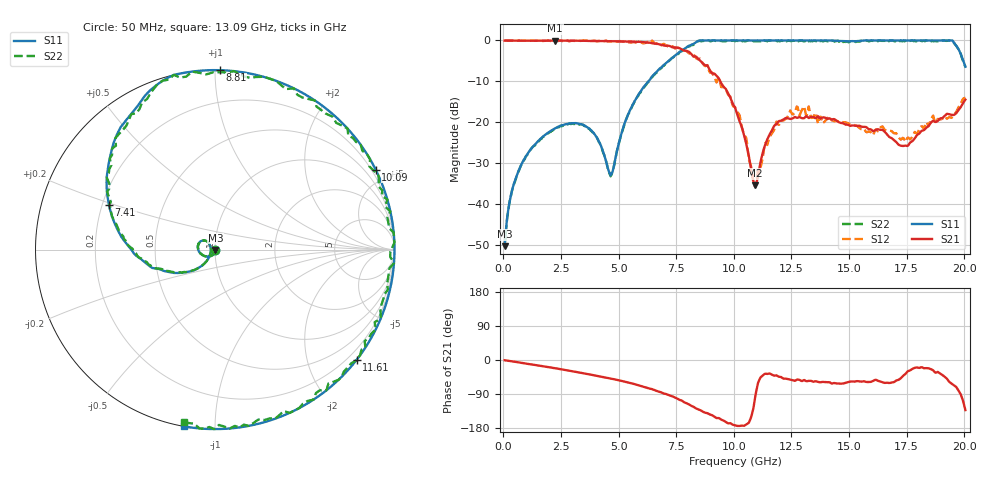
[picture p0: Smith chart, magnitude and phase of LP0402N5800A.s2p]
!	AVX	THIN	FILM	OPERATION
!	0402	SIZE	LOW	PASS	FILTER	P/N	LP0402N5800ANTR
!	Created	December	2017
!	Network	Analyzer	HP8720E	S.07.64:	"Feb23,"	2000	Serial	No.US39172382
#	MHz	S	dB	R	50
!	Frq	S11(dB)	S11(deg)	S21(dB)	S21(deg)	S12(dB)	S12(deg)	S22(dB)	S22(deg)
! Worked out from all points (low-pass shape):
!   501 points, 50 MHz to 20.05 GHz, reference 50 ohm
!   highest |S21| = -0.02 dB at 2.25 GHz (marker M1); lowest = -35.4 dB at 10.93 GHz (marker M2)
!   |S21| within 3 dB of the highest: start of sweep to 8.1 GHz
!   lowest |S11| = -50.2 dB at 50 MHz (marker M3), VSWR 1.01, Z = 50.3 - j0.14 ohm
!   |S11| at or under -10 dB: start of sweep to 6.287 GHz
!   |S22| runs from -50.2 to 0.0 dB; largest |S21 - S12| = 0.087
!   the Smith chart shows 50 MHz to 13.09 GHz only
!   S11 on the Smith chart (normalised r, x): 50 MHz: 1.01, -0.00; 7.41 GHz: 0.23, +0.19; 8.81 GHz: -0.00, +1.03; 10.09 GHz: -0.00, +4.26; 11.61 GHz: 0.00, -2.92; 13.09 GHz: 0.00, -0.84
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50  -50.17 -26.6  -0.03 -0.6  -0.02 -0.6  -50.17 -26.7
330  -37.57 -89.4  -0.04 -3.3  -0.02 -3.2  -37.77 -89.5
730  -30.84 -108.8  -0.04 -7.0  -0.07 -7.0  -30.84 -108.9
2250  -21.41 -166.0  -0.02 -21.7  0.00 -22.3  -21.41 -166.1
3410  -20.49 152.7  -0.08 -34.4  -0.05 -34.4  -20.49 152.7
4690  -32.50 -170.3  -0.19 -49.4  -0.19 -49.7  -32.70 -170.3
5410  -18.05 -130.4  -0.26 -59.2  -0.46 -59.6  -18.05 -130.5
6730  -7.13 -175.6  -0.89 -83.2  -0.59 -83.6  -7.23 -175.7
7410  -3.87 157.2  -1.70 -98.1  -1.76 -100.4  -3.87 157.0
8090  -1.22 125.7  -2.97 -118.7  -3.20 -120.4  -1.42 125.5
8810  0.00 88.5  -6.07 -139.8  -6.13 -145.1  -0.10 88.2
10050  0.00 28.4  -16.36 -172.5  -16.26 -172.9  -0.20 28.3
10090  0.00 26.4  -17.05 -173.1  -16.71 -170.0  -0.10 26.3
10930  0.00 -9.5  -35.36 -96.4  -35.82 -95.6  -0.20 -9.7
11610  0.00 -37.8  -22.35 -37.2  -23.00 -33.5  0.00 -38.0
13090  0.00 -100.0  -18.73 -54.2  -17.11 -63.7  -0.20 -100.2
13410  0.00 -111.9  -18.64 -56.4  -18.87 -61.6  -0.20 -111.9
14890  -0.19 -159.7  -20.53 -59.5  -20.05 -57.9  -0.29 -159.9
16730  0.00 148.1  -23.44 -60.7  -21.98 -72.4  -0.20 147.9
18450  0.00 82.1  -20.89 -21.8  -20.92 -14.7  -0.20 82.0
19490  -0.02 27.1  -18.16 -64.1  -18.59 -62.5  -0.22 26.9
20050  -6.42 8.1  -14.43 -132.2  -14.00 -140.9  -6.42 8.0
